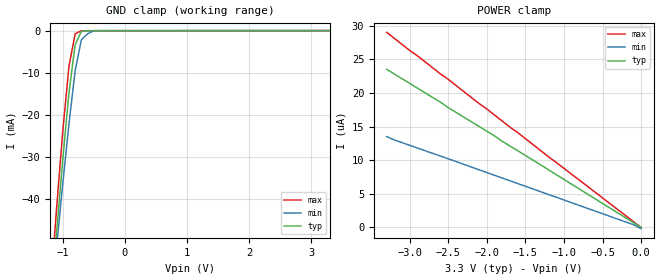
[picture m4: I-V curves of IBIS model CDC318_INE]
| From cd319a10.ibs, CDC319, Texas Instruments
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|   Model CDC318_INE
[Model]   CDC318_INE
Model_type   Input
Polarity   Non-Inverting
Vinl = 0.8V
Vinh = 2.0V
Vmeas = 1.5V
| variable   typ   min   max
C_comp   3.2p   NA   NA
[Voltage range]   3.3   3.135   3.465
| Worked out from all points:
|   GND clamp passes 1 mA (typ) near -0.73 V on its own axis
[GND_Clamp]
|  Voltage   I(typ)   I(min)   I(max)
-3.3V     -477mA     -423mA     -533mA
-1.2V     -66.6mA    -66.8mA    -62.4mA
-1.1V     -48.3mA    -51.6mA    -42.6mA
-1V       -30.8mA    -36.6mA    -24.1mA
-900mV    -14.9mA    -22.3mA    -8.56mA
-800mV    -3.36mA    -9.58mA    -750uA
-700mV    -202uA     -2.19mA    -51.3uA
-600mV    -33.2uA    -780uA     -36uA
-500mV    -27.3uA    -18.3uA    -34.8uA
3.3V      7.1pA      673nA      -1.45uA
[POWER_clamp]
|  Voltage   I(typ)   I(min)   I(max)
-3.3V     23.5uA     13.5uA     29uA
-3.2V     22.8uA     13uA       28.1uA
-100mV    714nA      408nA      878nA
0V        7.1pA      -186nA     7.32pA
